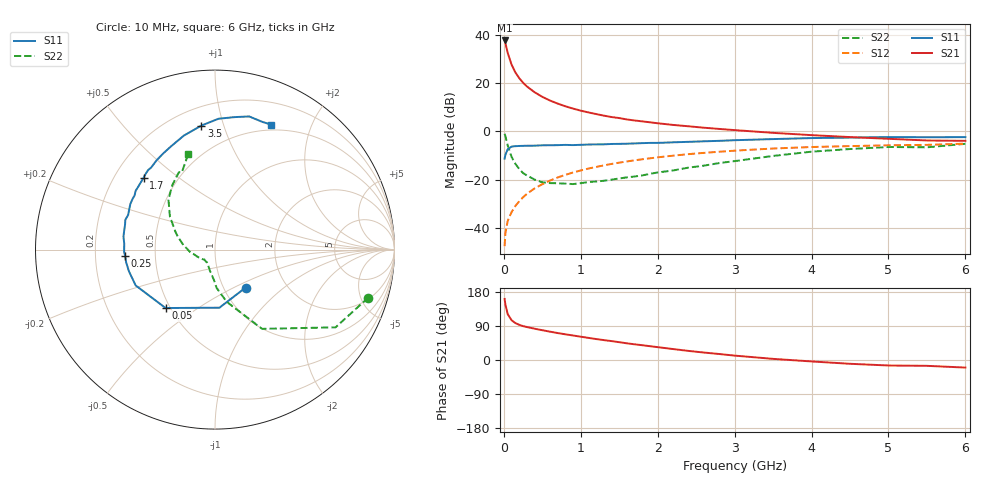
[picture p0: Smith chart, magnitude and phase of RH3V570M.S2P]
! SIEMENS Small Signal Semiconductors
! BFR106
! Si NPN RF Bipolar Junction Transistor in SOT23
! VCE = 3.5 V  IC = 70 mA
! Common Emitter S-Parameters:  August  1996
# GHz  S  MA  R  50
!  f  S11  S21  S12  S22
! GHz  MAG  ANG  MAG  ANG  MAG  ANG  MAG  ANG
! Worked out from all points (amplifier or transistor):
!   36 points, 10 MHz to 6 GHz, reference 50 ohm
!   highest |S21| = 37.9 dB at 10 MHz (marker M1)
!   |S21| within 3 dB of that: start of sweep to 34.09 MHz
!   unconditionally stable (mu >= 1): 204.1 MHz to 2.422 GHz
!   at 250 MHz: K = 1.03, MAG = 22.7 dB, |S12| = -27.4 dB
!   at 1.4 GHz: K = 1.06, MAG = 8.3 dB, |S12| = -13.5 dB
!   at 6 GHz: K = 0.99, MSG = 0.6 dB, |S12| = -5.1 dB
!   S11 on the Smith chart (normalised r, x): 10 MHz: 1.26, -0.58; 50 MHz: 0.47, -0.38; 250 MHz: 0.33, -0.03; 1.7 GHz: 0.32, +0.38; 3.5 GHz: 0.32, +0.84; 6 GHz: 0.44, +1.46
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0.01  0.2718 -51.2  78.56 161.2  0.0041 77.9  0.895 -17.4
0.02  0.3245 -85.6  69.25 146.6  0.0076 72.2  0.7994 -32.8
0.05  0.4263 -130.2  43.42 121.2  0.0137 62.4  0.5135 -59.3
0.1  0.4851 -155.7  24.8 105.0  0.0209 63.4  0.2972 -77.5
0.15  0.4947 -166.0  16.95 97.4  0.0282 67.5  0.2126 -87.7
0.2  0.5 -171.8  12.91 92.9  0.0353 70.6  0.1661 -92.5
0.25  0.5022 -176.2  10.34 89.4  0.0428 71.5  0.1362 -98.9
0.3  0.5063 -178.6  8.663 87.0  0.0504 72.8  0.1218 -103.3
0.4  0.507 176.1  6.561 82.6  0.0654 73.2  0.0998 -111.3
0.5  0.5152 171.9  5.263 78.6  0.0799 72.7  0.0876 -117.1
0.6  0.5169 168.1  4.412 74.8  0.0952 72.1  0.0843 -121.6
0.7  0.5199 164.6  3.812 71.1  0.1105 71.1  0.0837 -127.4
0.8  0.5264 161.6  3.346 67.8  0.1251 69.8  0.082 -132.9
1.1  0.5358 151.7  2.494 58.4  0.1692 65.8  0.0886 -143.8
1.4  0.5502 143.5  2 49.9  0.2112 61.3  0.0995 -154.0
1.7  0.5639 134.9  1.696 41.4  0.2512 56.6  0.1157 -165.4
2.2  0.5948 123.1  1.37 28.9  0.3141 48.5  0.1544 178.9
2.8  0.639 109.4  1.131 15.8  0.379 39.0  0.2203 160.6
3.5  0.695 96.3  0.937 3.0  0.4423 28.3  0.3101 144.0
4.5  0.7461 81.6  0.765 -10.0  0.4965 13.8  0.4315 123.4
5.5  0.7589 69.6  0.65 -15.4  0.5271 4.5  0.4684 113.2
6  0.7634 65.8  0.639 -20.0  0.559 -2.5  0.5535 105.6
